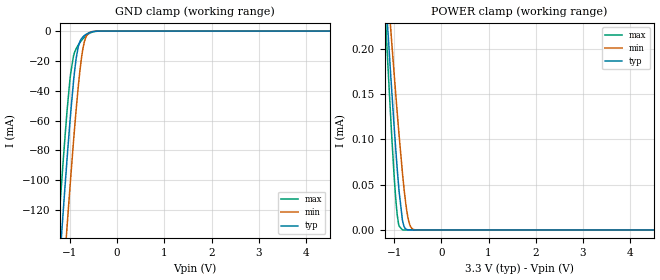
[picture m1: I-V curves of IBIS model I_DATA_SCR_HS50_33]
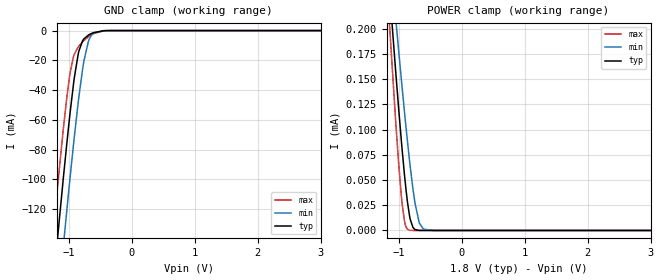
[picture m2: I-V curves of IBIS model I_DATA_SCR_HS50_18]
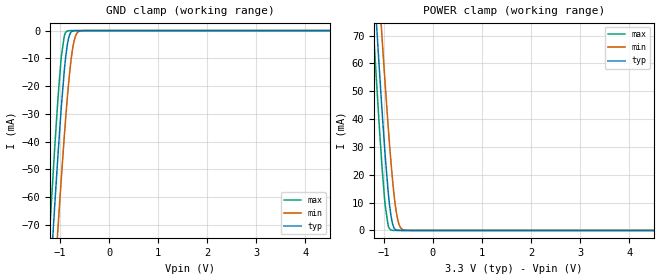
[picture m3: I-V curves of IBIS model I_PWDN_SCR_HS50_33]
| Texas Instruments Incorporated
| DS92LV0421
| 10-75MHz Channel Link II Serializer
| Marketing part#   Voltage Range   Package-type   Temperature
| DS92LV0421SQE   1.71V - 3.6V   36-Pin LLP   -40 to 105C
| DS92LV0421SQ   1.71V - 3.6V   36-Pin LLP   -40 to 105C
| DS92LV0421SQX   1.71V - 3.6V   36-Pin LLP   -40 to 105C
[IBIS Ver]   4.0
[File name]   ds92lv0421.ibs
[File Rev]   1.0
[Date]   03/27/2012
[Source]   Model built from TISPICE simulations at:
   Texas Instruments Incorporated.
   WEBENCH DESIGN CENTER
   12500 TI Blvd
   Dallas, TX -75243
   For Support e-mail: elab_scm_ibis@list.ti.com
[Notes]   Rev 1.0: 03/27/2012
   - Initial version of the IBIS model
   - All models are generated in Spectre
   - ccomp is listed in numerical order, for PVT information,
   please check notes above ccomp keyword for each model
   - All non-monotonic warnings can be ignored as per buffer behavior
[Disclaimer] This product is designed as an aid for customers of Texas Instruments.
   No warranties, either expressed or implied, with respect to this third
   party software (if any) or with respect to its fitness for any
   particular purpose is claimed by Texas Instruments or the author. The
   software (if any) is provided solely on an "as is" basis. The entire
   risk as to its quality and performance is with the customer
[Copyright]   (C)Copyright 2012 Texas Instruments Incorporated.
   All rights reserved.
|   DS92LV0421
[Component]  DS92LV0421
[Manufacturer]  Texas Instruments, Inc.
[Package]   | 36 pin LLP
|   typ   min   max
R_pkg   0   0   0
L_pkg   0   0   0
C_pkg   0   0   0
[Pin]   signal_name   model_name   R_pin   L_pin   C_pin
1   RxIN3-   I_DATA_SCR_HS50
2   RxIN3+   I_DATA_SCR_HS50
3   RES6   I_DATA_MC_HS50
4   ID[X]   NC
5   VDDL   POWER
6   SCL   IO_SMBUS_HS50
7   SDA   IO_SMBUS_HS50
8   RES0   NC
9   CONFIG[0]   I_DATA_SCR_HS50
10   CONFIG[1]   I_DATA_SCR_HS50
11   VDDP   POWER
12   RES1   NC
13   RES2   NC
14   VDDHS   POWER
15   DOUT-   NC
16   DOUT+   NC
17   VDDTX   POWER
18   RES3   NC
19   De-Emph   NC
20   VODSEL   I_DATA_SCR_HS50
21   BISTEN   I_DATA_SCR_HS50
22   VDDIO   POWER
23   PDB   I_PWDN_SCR_HS50
24   VDDRX   POWER
25   RES7   NC
26   MAPSEL   I_DATA_SCR_HS50
27   RES4   NC
28   RxIN0-   I_DATA_SCR_HS50
29   RxIN0+   I_DATA_SCR_HS50
30   RxIN1-   I_DATA_SCR_HS50
31   RxIN1+   I_DATA_SCR_HS50
32   RxIN2-   I_DATA_SCR_HS50
33   RxIN2+   I_DATA_SCR_HS50
34   RxClkIN-   I_DATA_SCR_HS50
35   RxClkIN+   I_DATA_SCR_HS50
36   RES5   NC
37   DAP   GND
[Package Model]   llp36_ds90ur907sq
[Diff pin]  inv_pin  vdiff  tdelay_typ  tdelay_min  tdelay_max
2   1   1.0   0.0s   0.0s   0.0s
29   28   1.0   0.0s   0.0s   0.0s
31   30   1.0   0.0s   0.0s   0.0s
33   32   1.0   0.0s   0.0s   0.0s
35   34   1.0   0.0s   0.0s   0.0s
[Model Selector]   I_DATA_SCR_HS50
I_DATA_SCR_HS50_33   I_DATA_SCR_HS50 input with VDD=3.3V
I_DATA_SCR_HS50_18   I_DATA_SCR_HS50 input with VDD=1.8V
[Model Selector]   I_DATA_MC_HS50
I_DATA_MC_HS50_33   I_DATA_MC_HS50 input with VDD=3.3V
I_DATA_MC_HS50_18   I_DATA_MC_HS50 input with VDD=1.8V
[Model Selector]   I_PWDN_SCR_HS50
I_PWDN_SCR_HS50_33   I_PWDN_SCR_HS50 input with VDD=3.3V
I_PWDN_SCR_HS50_18   I_PWDN_SCR_HS50 input with VDD=1.8V
[Model Selector]   IO_SMBUS_HS50
IO_SMBUS_HS50_33   IO_SMBUS_HS50 with VDD=3.3V
IO_SMBUS_HS50_18   IO_SMBUS_HS50 with VDD=1.8V
|   Package Model
[Define Package Model]  llp36_ds90ur907sq
[Manufacturer] Unknown
[OEM]  Unknown
[Description]  Package model with wirebonds at 3GHz
[Number Of Pins]  34
[Pin Numbers]
37   | 37 = DAP
1   | 1 = L1
2   | 2 = L2
3   | 3 = L3
4   | 4 = L4
5   | 5 = L5
6   | 6 = L6
7   | 7 = L7
8   | 8 = L8
9   | 9 = L9
10   | 10 = L10
11   | 11 = L11
12   | 12 = L12
13   | 13 = L13
14   | 14 = L14
15   | 15 = L15
16   | 16 = L16
17   | 17 = L17
19   | 19 = L19
20   | 20 = L20
21   | 21 = L21
22   | 22 = L22
23   | 23 = L23
24   | 24 = L24
25   | 25 = L25
26   | 26 = L26
28   | 28 = L28
29   | 29 = L29
30   | 30 = L30
31   | 31 = L31
32   | 32 = L32
33   | 33 = L33
34   | 34 = L34
35   | 35 = L35
[Model Data]
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[End Model Data]
[End Package Model]
| Models and submodels in the file (10): I_DATA_SCR_HS50_33 (Input), I_DATA_SCR_HS50_18 (Input), I_CLK_HS50_33 (Input), I_CLK_HS50_18 (Input), I_PWDN_SCR_HS50_33 (Input), I_PWDN_SCR_HS50_18 (Input), I_DATA_MC_HS50_18 (Input), I_DATA_MC_HS50_33 (Input), IO_SMBUS_HS50_33 (I/O_open_drain), IO_SMBUS_HS50_18 (I/O_open_drain)
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|   Model I_DATA_SCR_HS50_33
[Model] I_DATA_SCR_HS50_33
Model_type Input
Vinl =   0.8
Vinh =   2.0
|   typ   min   max
|   (nom)   (slow)   (fast)
C_comp   0.3665pF   0.3665pF   0.3665pF
[Temperature Range]   25.000   105.000   -40.000
[Voltage Range]   3.300V   3.0000V   3.6000V
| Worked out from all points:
|   GND clamp passes 1 mA (typ) near -0.58 V on its own axis
|   POWER clamp passes 1 mA (typ) near -2.02 V on its own axis
[GND Clamp]
|   Voltage   I(typ)   I(min)   I(max)
-3.3V     -1.166A    -1.209A    -1.134A
-1.32V    -202.1mA   -249mA     -167.1mA
-1.241V   -165.6mA   -212.4mA   -130.7mA
-1.142V   -121mA     -167.4mA   -86.89mA
-1.063V   -86.78mA   -132.3mA   -54.56mA
-983.4mV  -54.93mA   -98.36mA   -28.27mA
-924mV    -33.98mA   -74.16mA   -16.74mA
-825mV    -10.8mA    -38mA      -9.446mA
-755.7mV  -5.134mA   -18.34mA   -6.356mA
-696.3mV  -3.098mA   -7.601mA   -4.22mA
-567.6mV  -815.5uA   -746uA     -1.217mA
6.59V     0A         0A         0A
[POWER Clamp]
|   Voltage   I(typ)   I(min)   I(max)
-3.3V     2.159mA    1.892mA    2.559mA
-1.191V   270.3uA    306.6uA    243.1uA
-1.132V   220.6uA    264.4uA    182.9uA
-1.063V   164.1uA    216.1uA    115.7uA
-993.3mV  110.2uA    168.9uA    55.28uA
-933.9mV  67.72uA    129.8uA    16.89uA
-894.3mV  42.8uA     104.8uA    4.336uA
-825mV    11.61uA    64.2uA     166.8nA
-755.7mV  1.271uA    30.48uA    2.122nA
-696.3mV  130.3nA    11.15uA    0A
-557.7mV  0A         260.4nA    0A
6.59V     0A         0A         0A
|   Model I_DATA_SCR_HS50_18
[Model] I_DATA_SCR_HS50_18
Model_type Input
Vinl =   0.63
Vinh =   1.17
|   typ   min   max
|   (nom)   (fast)   (slow)
C_comp   0.5298pF   0.3665pF   0.5298pF
[Temperature Range]   25.000   105.000   -40.000
[Voltage Range]   1.800V   1.7100V   1.8900V
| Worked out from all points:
|   GND clamp passes 1 mA (typ) near -0.56 V on its own axis
[GND Clamp]
|   Voltage   I(typ)   I(min)   I(max)
-1.8V     -430.9mA   -477mA     -396.6mA
-1.238V   -164.5mA   -211.3mA   -129.6mA
-1.174V   -135.2mA   -181.7mA   -100.7mA
-1.093V   -99.54mA   -145.4mA   -66.37mA
-1.039V   -76.81mA   -121.8mA   -45.69mA
-984.6mV  -55.39mA   -98.86mA   -28.59mA
-930.6mV  -36.12mA   -76.78mA   -17.61mA
-855mV    -15.77mA   -48.21mA   -11.06mA
-763.2mV  -5.498mA   -20.14mA   -6.658mA
-687.6mV  -2.877mA   -6.556mA   -3.945mA
-450mV    -97.64uA   -77.9uA    -176.8uA
3.595V    0A         0A         0A
[POWER Clamp]
|   Voltage   I(typ)   I(min)   I(max)
-1.8V     803.7uA    754.7uA    897.4uA
-1.157V   241.8uA    282.5uA    208.5uA
-1.055V   157.9uA    210.7uA    108.4uA
-1.012V   124.1uA    181.2uA    70.17uA
-952.2mV  80.3uA     141.7uA    26.6uA
-914.4mV  55uA       117.4uA    9.25uA
-865.8mV  27.6uA     87.52uA    1.228uA
-822.6mV  10.92uA    62.89uA    149.1nA
-747mV    921.8nA    26.99uA    1.513nA
-682.2mV  75.41nA    8.215uA    0A
-612mV    3.441nA    1.296uA    0A
3.595V    0A         0A         0A
|   Model I_PWDN_SCR_HS50_33
[Model] I_PWDN_SCR_HS50_33
Model_type Input
Vinl =   0.8
Vinh =   2.0
|   typ   min   max
|   (nom)   (fast)   (slow)
C_comp   0.3665pF   0.3665pF   0.5298pF
[Temperature Range]   25.000   105.000   -40.000
[Voltage Range]   3.300V   3.0000V   3.6000V
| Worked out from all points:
|   GND clamp passes 1 mA (typ) near -0.79 V on its own axis
|   POWER clamp passes 1 mA (typ) near -0.79 V on its own axis
[GND Clamp]
|   Voltage   I(typ)   I(min)   I(max)
-3.3V     -740.6mA   -745.8mA   -738.2mA
-1.211V   -92.27mA   -118mA     -71.83mA
-1.191V   -86.5mA    -112.3mA   -65.95mA
-1.112V   -63.85mA   -90.11mA   -43.04mA
-1.043V   -44.84mA   -71.14mA   -24.45mA
-973.5mV  -27.25mA   -52.87mA   -9.257mA
-914.1mV  -14.38mA   -38.09mA   -1.938mA
-854.7mV  -5.279mA   -24.66mA   -158.3uA
-785.4mV  -769.6uA   -11.9mA    -11.81uA
-726mV    -91.41uA   -4.691mA   -6.467uA
-577.5mV  -3.449uA   -99.25uA   -4.919uA
6.59V     0A         0A         0A
[POWER Clamp]
|   Voltage   I(typ)   I(min)   I(max)
-3.3V     739mA      744.2mA    736.5mA
-1.211V   92.02mA    117.6mA    71.62mA
-1.191V   86.27mA    112mA      65.75mA
-1.112V   63.66mA    89.86mA    42.89mA
-1.043V   44.7mA     70.93mA    24.36mA
-973.5mV  27.14mA    52.7mA     9.21mA
-914.1mV  14.31mA    37.95mA    1.931mA
-854.7mV  5.248mA    24.55mA    164.4uA
-785.4mV  767.3uA    11.83mA    19.72uA
-726mV    94.5uA     4.66mA     14.93uA
-577.5mV  8.162uA    100.4uA    14.65uA
6.59V     0A         0A         0A
